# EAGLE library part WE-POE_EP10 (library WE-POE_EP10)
Transformer for Power-over-Ethernet WE-PoE - Flyback converter transducer particularly for PoE PDs - Insulation voltage 1,5 kVAC/1 min - Input voltages 36V till 80V -- Flyback converters -- Power-over-Ethernet PDs
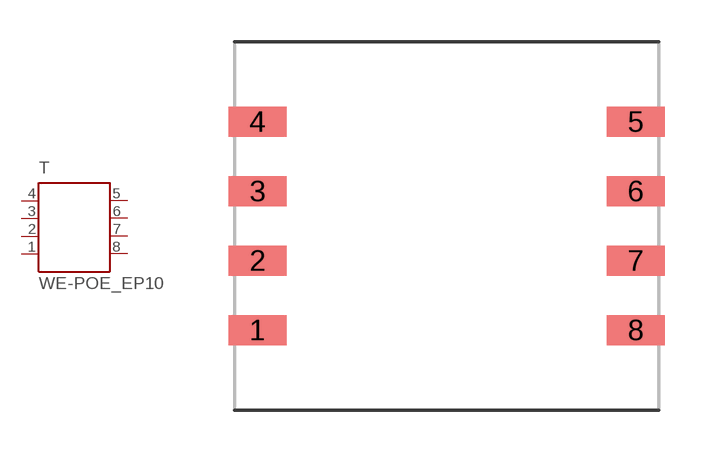
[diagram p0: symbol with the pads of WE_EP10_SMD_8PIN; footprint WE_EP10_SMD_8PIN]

Designator prefix T

## WE-POE_EP10, WE-POE_EP10-750310062 (MPN: 750310062; OC_FARNELL: 1849007; OC_NEWARK: 13T9826; PACKAGE: EP10; SUPPLIER: Wuerth Elektronik)  [WE_EP10_SMD_8PIN]
1  1  pas
2  2  pas
3  3  pas
4  4  pas
5  5  pas
6  6  pas
7  7  pas
8  8  pas

## Footprint WE_EP10_SMD_8PIN (pad centres in mm)
Transformer, EP10 SMD 8 Pin
smd 2.08 x 1.07: 1 -6.78,-3.735; 2 -6.78,-1.245; 3 -6.78,1.245; 4 -6.78,3.735; 5 6.78,3.735; 6 6.78,1.245; 7 6.78,-1.245; 8 6.78,-3.735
